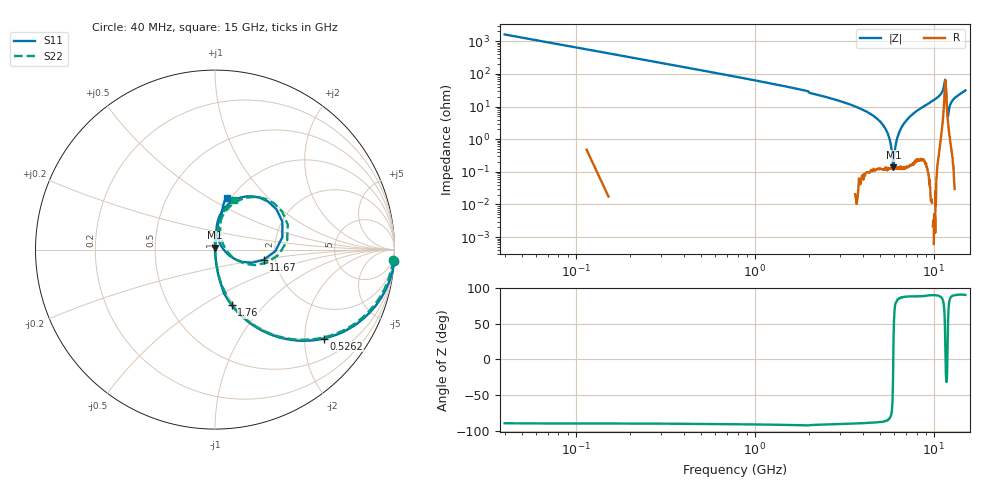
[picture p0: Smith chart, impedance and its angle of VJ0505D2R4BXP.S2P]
! VJ0505D2R4BXP
! MLCC placed on 25 mil thick microstrip substrate in series configuraton.
! DATE 06/29/2018  07:38
! CORRECTED  DATA
# GHz  S  MA  R  50.00
!  FREQ  S11M  S11A  S21M  S21A  S12M  S12A  S22M  S22A
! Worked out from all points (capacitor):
!   401 points, 40 MHz to 15 GHz, reference 50 ohm
!   read as one part in series: C = 2.45 pF near 114.8 MHz
!   lowest |Z| = 138 mohm at 5.949 GHz (marker M1)
!   series resonance near 5.933 GHz, so ESL is about 290 pH
!   S11 on the Smith chart (normalised r, x): 40 MHz: -1, -33; 526.2 MHz: 0.97, -2.47; 1.76 GHz: 0.98, -0.67; 11.67 GHz: 1.73, -0.21; 15 GHz: 0.96, +0.61
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0.04  1.001 -3.5  0.06178 86.2  0.06188 86.8  0.9942 -3.5
0.227  0.9488 -19.2  0.3299 70.9  0.33 70.9  0.9408 -19.1
0.5262  0.7824 -39.3  0.6344 51.4  0.635 51.4  0.7764 -39.2
1.0498  0.5225 -59.8  0.8657 31.6  0.8664 31.6  0.5196 -59.6
1.7604  0.3231 -73.3  0.9596 19.2  0.9598 19.2  0.3237 -73.3
2.5458  0.1826 -80.8  0.9865 11.1  0.9872 11.1  0.1832 -79.9
4.1914  0.06236 -85.2  0.9967 4.5  0.997 4.5  0.06247 -84.6
5.0516  0.02417 -87.7  0.9978 2.4  0.9984 2.4  0.02389 -83.4
5.4256  0.008457 -90.2  0.9981 1.6  0.9987 1.6  0.009021 -73.7
5.65  0.0006273 -108.5  0.9979 1.2  0.9987 1.2  0.002007 -9.3
5.7248  0.002783 102.9  0.998 1.0  0.9987 1.0  0.003584 49.3
5.837  0.006556 93.7  0.9982 0.8  0.9987 0.8  0.006842 70.9
5.9492  0.0108 93.8  0.9982 0.5  0.9982 0.6  0.01095 78.9
6.4728  0.02892 91.0  0.9977 -0.5  0.9982 -0.5  0.02882 84.1
7.52  0.06453 89.3  0.9954 -2.6  0.9961 -2.6  0.0655 83.5
10.0258  0.1637 84.1  0.9853 -8.6  0.9862 -8.6  0.1683 79.0
11.3722  0.3457 59.1  0.8535 -19.3  0.8546 -19.3  0.3602 54.4
11.5592  0.4064 22.6  0.6255 -12.6  0.6255 -12.6  0.4286 18.9
11.6714  0.2773 -11.9  0.7238 6.0  0.7242 6.0  0.2981 -14.2
11.9332  0.03979 30.1  0.9566 -0.5  0.9572 -0.5  0.05431 18.5
12.5316  0.1375 83.4  0.9851 -7.5  0.9858 -7.5  0.1425 77.9
15  0.2972 76.8  0.9554 -17.4  0.9553 -17.4  0.2979 69.1
